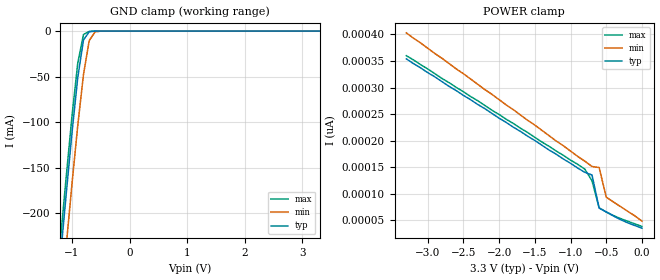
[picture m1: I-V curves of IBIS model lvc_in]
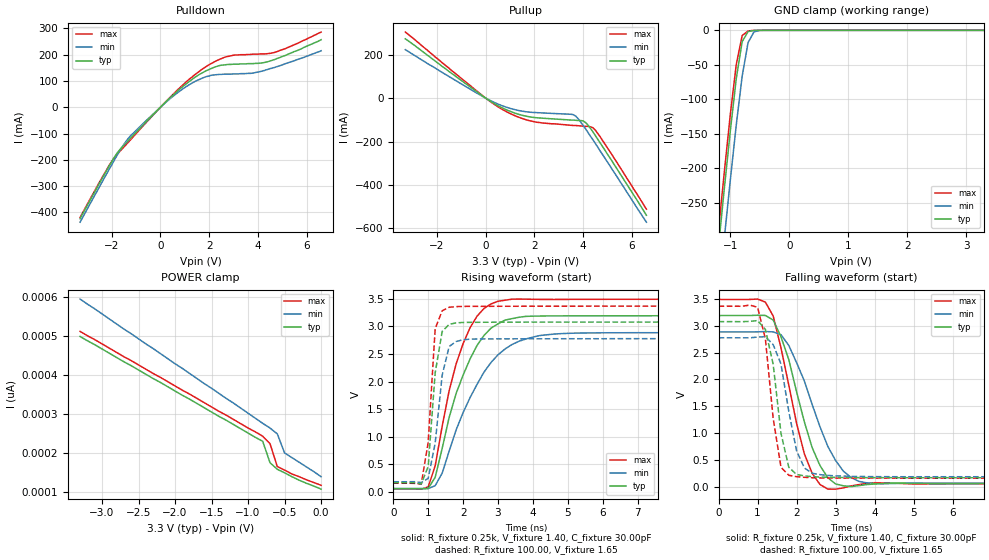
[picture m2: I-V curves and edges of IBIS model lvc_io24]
| IBIS file 16601x.ibs created by s2ibis2 version 1.1
| North Carolina State University Electronics Research Laboratory  1995
[IBIS ver]   2.1
[File name]   16601x.ibs
[File Rev]   1.0
[Date]   02/04/99 jbp
[Source]   Integrated Device Technology, Inc.
[Notes]   1.Temperatures: typ=25C, min=100C, max=0C 2.RRmp rates based
   on 50 ohm load.
[Disclaimer] Integrated Device Technology, Inc. ("IDT") hereby grants the
   user of this IBIS model a non-exclusive, nontransferable
   license to use this IBIS model under the following terms. The
   user is granted this license only to use the IBIS model and is
   not granted rights to sell, copy (except as needed to run the
   IBIS model), rent, lease or sub-license the IBIS model in
   whole or in part, or in modified form to anyone. The User may
   modify the IBIS model to suit its specific applications, but
   rights to derivative works and such modifications shall belong
   to IDT. This IBIS model is provided on an AS IS" basis and IDT
   makes absolutely no warranty with respect to the information
   contained herein. IDT DISCLAIMS AND CUSTOMER WAIVES ALL
   WARRANTIES, EXPRESS AND IMPLIED, INCLUDING WARRANTIES OF
   MERCHANTABILITY AND FITNESS FOR A PARTICULAR PURPOSE. THE
   ENTIRE RISK AS TO QUALITY AND PERFORMANCE IS WITH THE USER
   ACCORDINGLY, IN NO EVENT SHALL IDT BE LIABLE FOR ANY DIRECT OR
   INDIRECT DAMAGES, WHETHER IN CONTRACT OR TORT, INCLUDING ANY
   LOST PROFITS OR OTHER INCIDENTAL, CONSEQUENTIAL, EXEMPLARY, OR
   PUNITIVE DAMAGES ARISING OUT OF THE USE OR APPLICATION OF THE
   IBIS model. Further, IDT reserves the right to make changes
   without notice to any product herein to improve reliability,
   function, or design. IDT does not convey any license under
   patent rights or any other intellectual property rights,
   including those of third parties. IDT is not obligated to
   provide maintenance or support for the licensed IBIS model.
[Copyright]   Copyright 1997, Integrated Device Technology, Inc. all rights
   reserved
|   Component LVC16601
[Component]   LVC16601
[Manufacturer]   Integrated Device Technology
[Package]
| PA56
| variable   typ   min   max
R_pkg   6.50m   5.00m   10.00m
L_pkg   3.30nH   2.50nH   4.90nH
C_pkg   0.29pF   0.010pF   1.16pF
[Pin]  signal_name   model_name   R_pin   L_pin   C_pin
1   OEAB_   lvc_in
2   LEAB   lvc_in
3   A1   lvc_io24
4   GND   GND
5   A2   lvc_io24
6   A3   lvc_io24
7   VCC   POWER
8   A4   lvc_io24
9   A5   lvc_io24
10   A6   lvc_io24
11   GND   GND
12   A7   lvc_io24
13   A8   lvc_io24
14   A9   lvc_io24
15   A10   lvc_io24
16   A11   lvc_io24
17   A12   lvc_io24
18   GND   GND
19   A13   lvc_io24
20   A14   lvc_io24
21   A15   lvc_io24
22   VCC   POWER
23   A16   lvc_io24
24   A17   lvc_io24
25   GND   GND
26   A18   lvc_io24
27   OEBA_   lvc_in
28   LEBA   lvc_in
29   CLKENBA_   lvc_in
30   CLKBA   lvc_in
31   B18   lvc_io24
32   GND   GND
33   B17   lvc_io24
34   B16   lvc_io24
35   VCC   POWER
36   B15   lvc_io24
37   B14   lvc_io24
38   B13   lvc_io24
39   GND   GND
40   B12   lvc_io24
41   B11   lvc_io24
42   B10   lvc_io24
43   B9   lvc_io24
44   B8   lvc_io24
45   B7   lvc_io24
46   GND   GND
47   B6   lvc_io24
48   B5   lvc_io24
49   B4   lvc_io24
50   VCC   POWER
51   B3   lvc_io24
52   B2   lvc_io24
53   GND   GND
54   B1   lvc_io24
55   CLKAB   lvc_in
56   CLKENAB_   lvc_in
| Models and submodels in the file (2): lvc_in (Input), lvc_io24 (I/O)
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| in   in   dummy_model
| oe   oe
|   Model lvc_in
[Model]   lvc_in
Model_type   Input
Vinl =  0.800V
Vinh =  2.000V
C_comp   3.00pF   NA   NA
[Temperature Range]   25.00   100.00   0.000
[Voltage Range]   3.30V   3.00V   3.60V
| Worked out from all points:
|   GND clamp passes 1 mA (typ) near -0.70 V on its own axis
[GND_clamp]
| voltage   I(typ)   I(min)   I(max)
-3.3V     -1.806A    -1.858A    -1.789A
-1.2V     -248mA     -306mA     -229mA
-1.1V     -179mA     -236mA     -160mA
-1V       -112mA     -168mA     -93.56mA
-900mV    -51.39mA   -104mA     -35.36mA
-800mV    -9.697mA   -47.7mA    -3.786mA
-700mV    -714uA     -10.4mA    -348uA
-600mV    -52.42uA   -951uA     -8.225uA
-500mV    -126nA     -30.48uA   -10.89nA
3.3V      34.69pA    75.27pA    23pA
[POWER_clamp]
| voltage   I(typ)   I(min)   I(max)
-3.3V     354pA      403pA      360pA
-800mV    140pA      161pA      146pA
-700mV    135pA      151pA      124pA
-600mV    72.75pA    149pA      72.79pA
-500mV    65.09pA    93.05pA    65.39pA
-300mV    50.77pA    75.27pA    52.78pA
0V        34.68pA    47.91pA    37.83pA
|   Model lvc_io24
[Model]   lvc_io24
Model_type   I/O
Polarity   Non-Inverting
Enable   Active-High
Vinl =  0.000V
Vinh =  2.000V
Vmeas =  1.500V
C_comp   3.00pF   NA   NA
[Temperature Range]   25.00   100.00   0.000
[Voltage Range]   3.30V   3.00V   3.60V
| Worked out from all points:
|   slope of the pulldown table from 0 to 0.495 V, typ, clamps not added: 11.1 ohm
|   slope of the pullup table from 0 to 0.495 V, typ, clamps not added: 14.5 ohm
|   GND clamp passes 1 mA (typ) near -0.65 V on its own axis
|   rising waveform, R_fixture 0.25k, V_fixture 1.40, C_fixture 30.00pF: 20-80 % time 967ps typ, 1.23ns min, 806ps max; typ from 0.061 V to 3.19 V
|   rising waveform, R_fixture 100.00, V_fixture 1.65: 20-80 % time 256ps typ, 312ps min, 204ps max; typ from 0.171 V to 3.08 V
|   falling waveform, R_fixture 0.25k, V_fixture 1.40, C_fixture 30.00pF: 20-80 % time 717ps typ, 899ps min, 627ps max; typ from 3.19 V to 0.061 V
|   falling waveform, R_fixture 100.00, V_fixture 1.65: 20-80 % time 344ps typ, 384ps min, 299ps max; typ from 3.08 V to 0.171 V
[Pulldown]
| voltage   I(typ)   I(min)   I(max)
-3.3V     -424mA     -437mA     -419mA
-2.1V     -222mA     -235mA     -220mA
-1.8V     -177mA     -186mA     -182mA
-1.4V     -135mA     -128mA     -141mA
47.68nV   4.5nA      4.1nA      4.75nA
900mV     77.5mA     68.6mA     83.2mA
1.8V      135mA      114mA      150mA
2.6V      161mA      126mA      189mA
3.7V      166mA      129mA      201mA
4.4V      173mA      144mA      204mA
5.1V      196mA      165mA      222mA
6.6V      257mA      215mA      286mA
[Pullup]
| voltage   I(typ)   I(min)   I(max)
-3.3V     273mA      223mA      304mA
-200mV    15.7mA     12.6mA     17.8mA
800mV     -51.2mA    -39.9mA    -59.2mA
1.4V      -75.9mA    -58mA      -89.7mA
2V        -89.2mA    -66.1mA    -109mA
3.5V      -101mA     -74.3mA    -125mA
3.7V      -102mA     -83mA      -126mA
4.1V      -112mA     -141mA     -130mA
4.4V      -155mA     -191mA     -136mA
4.5V      -172mA     -208mA     -147mA
5.2V      -292mA     -329mA     -263mA
6.6V      -539mA     -571mA     -511mA
[GND_clamp]
| voltage   I(typ)   I(min)   I(max)
-3.3V     -2.216A    -2.282A    -2.195A
-1.2V     -312mA     -384mA     -288mA
-1.1V     -227mA     -299mA     -203mA
-1V       -145mA     -216mA     -121mA
-900mV    -69.82mA   -137mA     -49.38mA
-800mV    -16.36mA   -66.43mA   -7.569mA
-700mV    -1.849mA   -17.78mA   -961uA
-600mV    -147uA     -2.322mA   -22.41uA
-500mV    -324nA     -78.01uA   -27.71nA
3.3V      107pA      176pA      95.6pA
[POWER_clamp]
| voltage   I(typ)   I(min)   I(max)
-3.3V     499pA      595pA      512pA
-800mV    230pA      276pA      243pA
-700mV    175pA      264pA      224pA
-600mV    158pA      249pA      165pA
-500mV    149pA      200pA      156pA
-400mV    139pA      188pA      146pA
0V        107pA      139pA      117pA
[Ramp]
| variable   typ   min   max
dV/dt_r   1.45/0.32n   1.21/0.34n   1.64/0.23n
dV/dt_f   1.59/0.39n   1.41/0.50n   1.76/0.35n
R_load = 50.00
[Rising Waveform]
R_fixture = 0.25k
V_fixture = 1.40
C_fixture = 30.00pF
R_dut = 7.00m
L_dut = 3.30nH
C_dut = 0.29pF
| time   V(typ)   V(min)   V(max)
0s        61.33mV    67.59mV    57.9mV
1ns       68.22mV    64.57mV    95.17mV
1.2ns     268mV      117mV      475mV
1.4ns     789mV      343mV      1.189V
1.6ns     1.351V     741mV      1.833V
2ns       2.115V     1.438V     2.684V
2.4ns     2.652V     1.949V     3.181V
3ns       3.042V     2.482V     3.45V
5ns       3.187V     2.87V      3.484V
19.8ns    3.189V     2.884V     3.487V
[Rising Waveform]
R_fixture = 100.00
V_fixture = 1.65
R_dut = 7.00m
L_dut = 3.30nH
C_dut = 0.29pF
| time   V(typ)   V(min)   V(max)
0s        171mV      188mV      162mV
800ps     146mV      174mV      143mV
1ns       466mV      249mV      904mV
1.2ns     2.157V     886mV      2.955V
1.4ns     2.905V     2.113V     3.279V
1.6ns     3.033V     2.632V     3.342V
1.8ns     3.06V      2.723V     3.353V
2ns       3.067V     2.755V     3.357V
2.6ns     3.071V     2.77V      3.359V
19.8ns    3.075V     2.775V     3.362V
[Falling Waveform]
R_fixture = 0.25k
V_fixture = 1.40
C_fixture = 30.00pF
R_dut = 7.00m
L_dut = 3.30nH
C_dut = 0.29pF
| time   V(typ)   V(min)   V(max)
0s        3.189V     2.884V     3.487V
1.2ns     3.19V      2.891V     3.438V
1.4ns     3.105V     2.884V     3.179V
1.6ns     2.792V     2.831V     2.586V
2.2ns     1.208V     1.968V     614mV
2.4ns     729mV      1.532V     251mV
2.8ns     171mV      754mV      -40.63mV
3.4ns     6.014mV    174mV      19.04mV
4ns       54.32mV    61.62mV    77.9mV
19.8ns    61.33mV    67.6mV     57.91mV
[Falling Waveform]
R_fixture = 100.00
V_fixture = 1.65
R_dut = 7.00m
L_dut = 3.30nH
C_dut = 0.29pF
| time   V(typ)   V(min)   V(max)
0s        3.075V     2.775V     3.362V
1ns       3.095V     2.788V     3.342V
1.2ns     2.93V      2.794V     2.754V
1.4ns     2.278V     2.646V     1.271V
1.6ns     995mV      2.286V     365mV
1.8ns     365mV      1.403V     216mV
2ns       230mV      672mV      190mV
2.2ns     205mV      352mV      178mV
2.8ns     178mV      214mV      165mV
19.8ns    171mV      188mV      162mV
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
